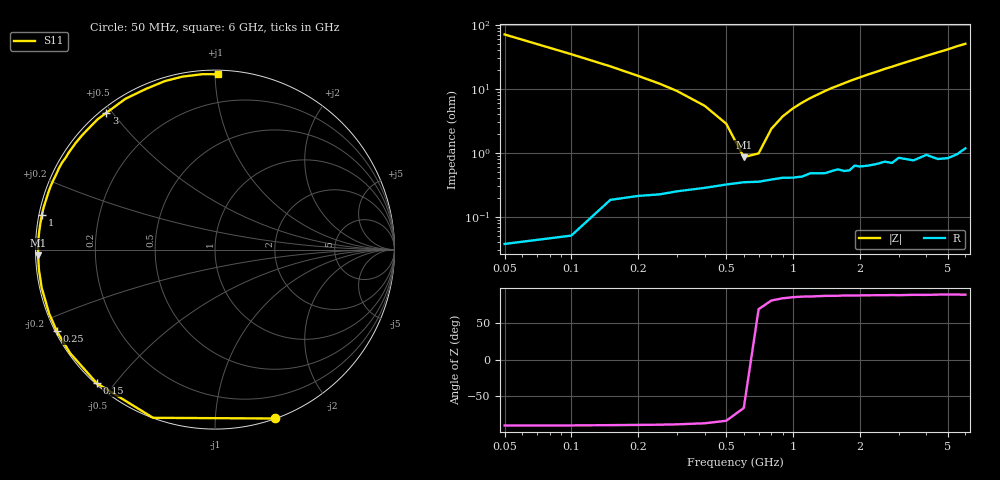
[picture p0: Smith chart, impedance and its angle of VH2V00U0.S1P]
! Infineon Technologies  Discrete & RF Semiconductors
! BB 814
! Si Tuning Diode in SOT23
! VR = 2 V
! S-Parameters:  July  1999
# GHz  S  MA  R  50
!  f  S11
! GHz  MAG  ANG
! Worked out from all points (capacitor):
!   34 points, 50 MHz to 6 GHz, reference 50 ohm
!   read as one part to ground: C = 44.6 pF near 50 MHz
!   lowest |Z| = 859 mohm at 600 MHz (marker M1)
!   series resonance near 646.2 MHz, so ESL is about 1.4 nH
!   S11 on the Smith chart (normalised r, x): 50 MHz: 0.00, -1.42; 150 MHz: 0.00, -0.45; 250 MHz: 0.00, -0.24; 1 GHz: 0.01, +0.10; 3 GHz: 0.02, +0.48; 6 GHz: 0.02, +1.02
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0.05  0.9995 -70.3
0.1  0.9986 -110.2
0.15  0.9939 -131.5
0.2  0.9923 -144.5
0.25  0.9916 -152.8
0.3  0.9903 -159.0
0.4  0.9888 -167.6
0.5  0.9873 -173.5
0.6  0.9862 -178.2
0.7  0.9859 177.9
0.8  0.9848 174.6
1  0.9839 168.7
1.2  0.9814 163.6
1.4  0.9815 158.9
1.6  0.9791 154.6
1.8  0.9802 150.3
2  0.9778 146.4
2.2  0.9775 142.5
2.4  0.9766 139.0
2.6  0.9754 135.2
2.8  0.977 132.0
3  0.9732 128.5
3.5  0.9772 120.7
4  0.9744 113.3
4.5  0.9796 106.6
5  0.9806 100.6
5.5  0.9798 94.2
6  0.977 89.1
